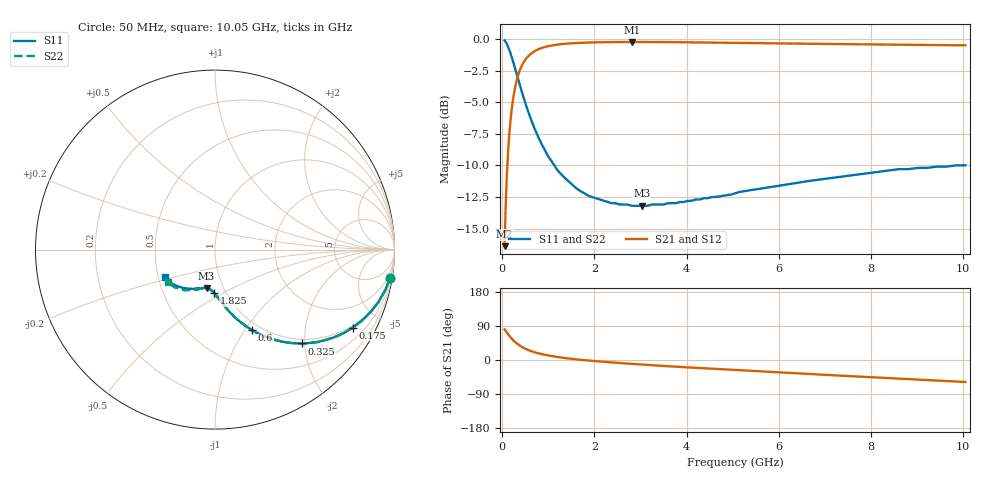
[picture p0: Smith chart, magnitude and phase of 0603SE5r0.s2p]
! AVX Thin Film Operation		Date: August 2001
! Description: Accu-P® Series, Thin Film, SMD, RF Capacitor
! Part Number: 06035J5R0ABT
! 50 MHz  -  10.05 GHz
! Serial Measurements
# mhz S db R 50
!	S11		S21		S12		S22
!	dB	Phase	dB	Phase	dB	Phase	dB	Phase
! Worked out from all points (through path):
!   401 points, 50 MHz to 10.05 GHz, reference 50 ohm
!   highest |S21| = -0.22 dB at 2.825 GHz (marker M1); lowest = -16.4 dB at 50 MHz (marker M2)
!   group delay of S21, straight-line fit = 23.7 ps
!   lowest |S11| = -13.2 dB at 3.025 GHz (marker M3), VSWR 1.56, Z = 41.7 - j18.7 ohm
!   |S11| at or under -10 dB: 1.131 GHz to 9.85 GHz (8.719 GHz wide, 159 % of centre)
!   |S22| runs from -13.2 to -0.1 dB; largest |S21 - S12| = 0
!   S11 on the Smith chart (normalised r, x): 50 MHz: 1, -12; 175 MHz: 0.91, -3.58; 325 MHz: 0.91, -1.94; 600 MHz: 0.91, -1.08; 1.825 GHz: 0.88, -0.45; 10.05 GHz: 0.54, -0.19
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50  -0.10 -9.1  -16.40 80.9  -16.40 80.9  -0.10 -9.1
75  -0.22 -13.5  -13.01 76.5  -13.01 76.5  -0.22 -13.5
125  -0.59 -21.9  -8.94 68.1  -8.94 68.1  -0.59 -21.9
175  -1.09 -29.5  -6.55 60.5  -6.55 60.5  -1.09 -29.5
250  -1.98 -39.2  -4.38 50.8  -4.38 50.8  -1.98 -39.2
325  -2.93 -47.1  -3.09 42.9  -3.09 42.9  -2.93 -47.1
375  -3.57 -51.5  -2.52 38.4  -2.52 38.4  -3.57 -51.5
450  -4.49 -57.1  -1.91 32.9  -1.91 32.9  -4.49 -57.1
600  -6.13 -65.3  -1.22 24.7  -1.22 24.7  -6.13 -65.2
775  -7.71 -72.0  -0.81 17.9  -0.81 17.9  -7.71 -72.0
1000  -9.31 -78.2  -0.55 11.8  -0.55 11.8  -9.31 -78.1
1275  -10.69 -83.4  -0.40 6.6  -0.40 6.6  -10.69 -83.2
1725  -12.10 -89.8  -0.28 0.2  -0.28 0.2  -12.10 -89.5
1825  -12.32 -90.9  -0.27 -0.9  -0.27 -0.9  -12.26 -90.5
2350  -12.97 -96.3  -0.23 -6.2  -0.23 -6.2  -12.97 -95.7
2825  -13.20 -101.0  -0.22 -10.4  -0.22 -10.4  -13.20 -99.7
3025  -13.20 -102.5  -0.22 -12.1  -0.22 -12.1  -13.20 -101.5
3400  -13.10 -105.0  -0.23 -14.9  -0.23 -14.9  -13.10 -104.0
5050  -12.22 -117.4  -0.28 -26.6  -0.28 -26.6  -12.16 -115.4
6725  -11.20 -129.0  -0.36 -37.3  -0.36 -37.3  -11.20 -125.0
8400  -10.39 -140.1  -0.44 -47.9  -0.44 -47.9  -10.39 -135.1
10050  -9.99 -150.8  -0.48 -58.0  -0.48 -58.0  -9.96 -144.8
